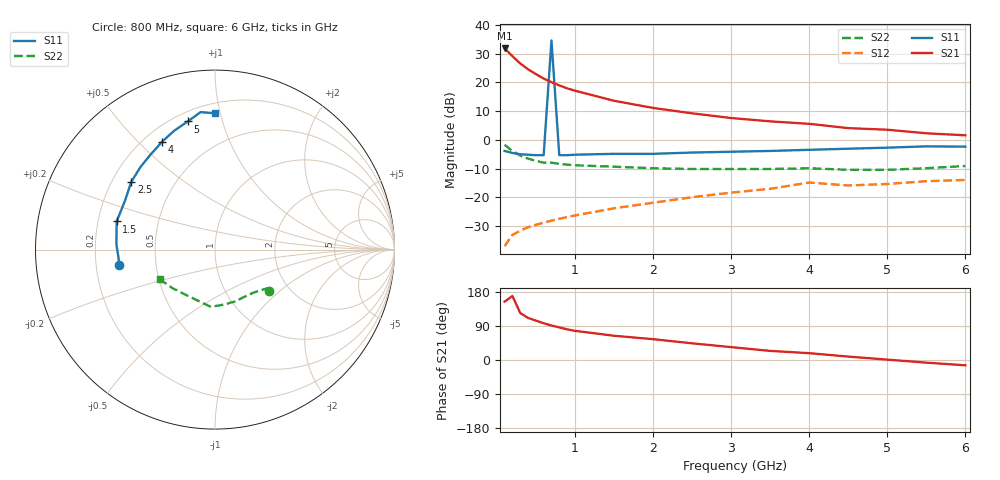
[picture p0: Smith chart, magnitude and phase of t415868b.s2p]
!AT-41586
!S-PARAMETERS at Vce=8V Ic=25mA. LAST UPDATED 08-03-92
# ghz s ma r 50
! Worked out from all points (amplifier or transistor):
!   20 points, 100 MHz to 6 GHz, reference 50 ohm
!   highest |S21| = 31.9 dB at 100 MHz (marker M1)
!   |S21| within 3 dB of that: start of sweep to 209.7 MHz
!   unconditionally stable (mu >= 1): 1.905 GHz to 2.149 GHz
!   at 400 MHz: K = 0.55, MSG = 27.5 dB, |S12| = -30.5 dB
!   at 1.5 GHz: K = 0.93, MSG = 18.8 dB, |S12| = -23.9 dB
!   at 6 GHz: K = 0.85, MSG = 7.8 dB, |S12| = -14.0 dB
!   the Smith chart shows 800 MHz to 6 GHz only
!   S11 on the Smith chart (normalised r, x): 800 MHz: 0.30, -0.07; 1.5 GHz: 0.28, +0.13; 2.5 GHz: 0.28, +0.33; 4 GHz: 0.27, +0.59; 5 GHz: 0.25, +0.78; 6 GHz: 0.27, +0.96
0.1  0.64 -61.0  39.4 154.0  0.014 64.0  0.82 -24.0
0.2  0.59 -101.0  28.7 169.0  0.022 53.0  0.64 -35.0
0.3  0.56 -125.0  21.4 124.0  0.026 49.0  0.53 -38.0
0.4  0.55 -140.0  17 111.0  0.03 49.0  0.47 -39.0
0.5  0.54 -151.0  14 104.0  0.033 50.0  0.43 -38.0
0.6  0.54 -159.0  11.7 97.0  0.036 52.0  0.4 -38.0
0.7  54 -166.0  10.1 91.0  0.039 53.0  0.4 -37.0
0.8  0.54 -171.0  8.9 86.0  0.042 55.0  0.38 -37.0
0.9  0.54 -176.0  7.9 81.0  0.045 56.0  0.37 -37.0
1  0.55 177.0  7.2 77.0  0.048 57.0  0.36 -37.0
1.5  0.57 164.0  4.8 64.0  0.064 59.0  0.34 -42.0
2  0.57 152.0  3.6 55.0  0.08 57.0  0.32 -49.0
2.5  0.6 141.0  2.9 44.0  0.1 55.0  0.31 -58.0
3  0.62 132.0  2.4 34.0  0.12 52.0  0.31 -68.0
3.5  0.64 124.0  2.1 24.0  0.14 49.0  0.31 -80.0
4  0.67 116.0  1.9 18.0  0.18 45.0  0.32 -94.0
4.5  0.7 109.0  1.6 9.0  0.16 45.0  0.3 -109.0
5  0.73 102.0  1.5 1.0  0.17 42.0  0.3 -123.0
5.5  0.77 96.0  1.3 -7.0  0.19 38.0  0.32 -138.0
6  0.76 90.0  1.2 -14.0  0.2 33.0  0.35 -152.0
